// TwinCAT 3 PLC project mc
// ProgramVersion: 3.1.0.9
// libraries:
//   Tc2_MC2, * (Beckhoff Automation GmbH)
//   Tc2_Standard, * (Beckhoff Automation GmbH)
//   Tc2_System, * (Beckhoff Automation GmbH)
//   Tc3_Interfaces, * (Beckhoff Automation GmbH)
//   Tc3_Module, * (Beckhoff Automation GmbH)
// project tree:
//   / PlcTask.TcTTO
//   POUs/ MAIN.TcPOU
// real-time tasks:
//   TASK PlcTask: cycle T#10ms, priority 20, ADS port 350
// motion (NC):
//   TASK NC-Task 1 SAF: cycle T#2ms, priority 4, ADS port 501
//   TASK NC-Task 1 SVB: cycle T#10ms, priority 8, ADS port 511
//   AXIS Axis 1 (id 1)
//     OtherSettings: AllowMotionCmdToSlave=true
//     encoder EncType=8
//       EncPara: MaxCount=#x0036ee7f
//     drive DrvType=9
//       DrvPara: MaxCount=#xffffffff, DriveControlDWord=#x00030000
//         Analog: VeloScale=6
//         TimeComp: TaskDelayCycles=1
//     controller CtrType=1
//       CtrPara: PriorControlFactor=1
//         PosDiffControl: Enable=false, Range=10
//         Observer: BandWidth=20
//   AXIS Axis 2 (id 2)
//     OtherSettings: AllowMotionCmdToSlave=true
//     encoder EncType=8
//       EncPara: MaxCount=#x0036ee7f
//     drive DrvType=9
//       DrvPara: MaxCount=#xffffffff, DriveControlDWord=#x00030000
//         Analog: VeloScale=6
//         TimeComp: TaskDelayCycles=1
//     controller CtrType=1
//       CtrPara: PriorControlFactor=1
//         PosDiffControl: Enable=false
//         Observer: BandWidth=20
// I/O:
//   DEVICE Device 1 (EtherCAT), AmsNetId 5.18.64.212.2.1
//     Term 1 (EK1200) [EK1200-5000 EtherCAT Power supply (2A E-Bus)]
//       Term 2 (EL1004) [EL1004 4Ch. Dig. Input 24V, 3ms]
//       Term 3 (EL2024) [EL2024 4Ch. Dig. Output 24V, 2A]
//       Term 4 (EL9011) [EL9011 End Terminal]
//   DEVICE Device 4 (EtherCAT), AmsNetId 5.18.64.212.5.1
//     Drive 5 (AX5203-0000-0011) [AX5203-0000 EtherCAT Drive (SoE, 2 Ch.)]
//   DEVICE Device 3 (USB)
//     Box 7 (CX2100 Power Supply)
//   DEVICE Device 5 (NOV-DP-RAM)
// variable links:
//   NC-Task 1 SAF/Axes/Axis 1 <-> Device 4 (EtherCAT)/Drive 5 (AX5203-0000-0011)
//     Drive/Inputs/In/nDcOutputTime <-> InfoData/DcOutputShift
//     Drive/Inputs/In/nState1 <-> AT 1/Drive status word @bit 8
//     Drive/Inputs/In/nState2 <-> AT 1/Drive status word
//     Drive/Inputs/In/nState4 @bit 1 <-> WcState/InputToggle
//     Drive/Inputs/In/nState4 <-> WcState/WcState
//     Drive/Outputs/Out/nCtrl1 <-> MDT 1/Master control word @bit 8
//     Drive/Outputs/Out/nDataOut2 <-> MDT 1/Velocity command value
//     Enc/Inputs/In/nDataIn1 <-> AT 1/Position feedback 1 value
//     Enc/Inputs/In/nDcInputTime <-> InfoData/DcInputShift
//     Enc/Inputs/In/nState4 @bit 1 <-> WcState/InputToggle
//     Enc/Inputs/In/nState4 <-> WcState/WcState
//   NC-Task 1 SAF/Axes/Axis 2 <-> Device 4 (EtherCAT)/Drive 5 (AX5203-0000-0011)
//     Drive/Inputs/In/nDcOutputTime <-> InfoData/DcOutputShift
//     Drive/Inputs/In/nState1 <-> AT 2/Drive status word @bit 8
//     Drive/Inputs/In/nState2 <-> AT 2/Drive status word
//     Drive/Inputs/In/nState4 @bit 1 <-> WcState/InputToggle
//     Drive/Inputs/In/nState4 <-> WcState/WcState
//     Drive/Outputs/Out/nCtrl1 <-> MDT 2/Master control word @bit 8
//     Drive/Outputs/Out/nDataOut2 <-> MDT 2/Velocity command value
//     Enc/Inputs/In/nDataIn1 <-> AT 2/Position feedback 1 value
//     Enc/Inputs/In/nDcInputTime <-> InfoData/DcInputShift
//     Enc/Inputs/In/nState4 @bit 1 <-> WcState/InputToggle
//     Enc/Inputs/In/nState4 <-> WcState/WcState
//   mc/mc Instance <-> NC-Task 1 SAF/Axes/Axis 1
//     PlcTask Inputs/MAIN.axis1.NcToPlc <-> Outputs/ToPlc
//     PlcTask Outputs/MAIN.axis1.PlcToNc <-> Inputs/FromPlc

CONFIGURATION mc
    RESOURCE PLC ON TwinCAT3
        TASK PlcTask(INTERVAL := T#10ms, PRIORITY := 20);
        PROGRAM MAIN WITH PlcTask : MAIN;
    END_RESOURCE
END_CONFIGURATION

// ---- POUs/MAIN.TcPOU
PROGRAM MAIN
VAR
	power1:MC_Power;
	axis1: AXIS_REF;
	power_do: BOOL;
	jog1:MC_Jog;
	jog_for: BOOL;
	jog_back: BOOL;
	gearin:mc_gearin;
	gearout:mc_gearout;
	power2:mc_power;
	axis2:axis_ref;
	gearin_do:BOOL;
	gearout_do:bool;
END_VAR

power1(
	Axis:=axis1 , 
	Enable:=power_do , 
	Enable_Positive:=TRUE , 
	Enable_Negative:= TRUE, 
	Override:= , 
	BufferMode:= , 
	Options:= , 
	Status=> , 
	Busy=> , 
	Active=> , 
	Error=> , 
	ErrorID=> );
jog1(
	Axis:=axis1 , 
	JogForward:=jog_for , 
	JogBackwards:= jog_back, 
	Mode:= , 
	Position:= , 
	Velocity:= , 
	Acceleration:= , 
	Deceleration:= , 
	Jerk:= , 
	Done=> , 
	Busy=> , 
	Active=> , 
	CommandAborted=> , 
	Error=> , 
	ErrorID=> );
gearin(
	Master:= axis1, 
	Slave:=axis2 , 
	Execute:= gearin_do, 
	RatioNumerator:=1 , 
	RatioDenominator:=1 , 
	Acceleration:= , 
	Deceleration:= , 
	Jerk:= , 
	BufferMode:= , 
	Options:= , 
	InGear=> , 
	Busy=> , 
	Active=> , 
	CommandAborted=> , 
	Error=> , 
	ErrorID=> );
gearout(
	Slave:=axis2 , 
	Execute:=gearout_do , 
	Options:= , 
	Done=> , 
	Busy=> , 
	Error=> , 
	ErrorID=> );

END_PROGRAM
